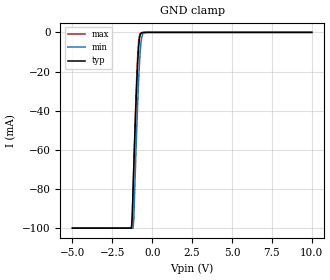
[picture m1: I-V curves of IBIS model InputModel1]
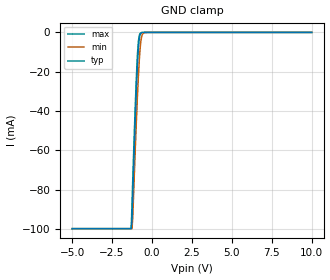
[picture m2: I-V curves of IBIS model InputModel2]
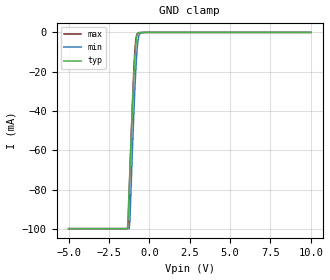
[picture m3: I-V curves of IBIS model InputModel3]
[IBIS Ver]   2.1
[File name]   pa200bv5.ibs   | pa= PSOP, f200bv= abbr chip name, 5= 5V Vcc
[File Rev]   2.00
[Date]   28-February-96
[Source]   File generated from lab measurements at Intel Corporation
[Notes]   Rev 2.00 All data was replaced by actual measurements
   performed in a lab.
[Disclaimer] INTEL DEVELOPER'S SOFTWARE LICENSE AGREEMENT
| BY USING THIS SOFTWARE, YOU ARE AGREEING TO BE BOUND
| BY THE TERMS OF THIS AGREEMENT.  DO NOT USE THE SOFTWARE
| UNTIL YOU HAVE CAREFULLY READ AND AGREED TO THE FOLLOWING
| TERMS AND CONDITIONS.  IF YOU DO NOT AGREE TO THE TERMS
| OF THIS AGREEMENT, PROMPTLY RETURN THE SOFTWARE PACKAGE
| AND ANY ACCOMPANYING ITEMS.
| IF YOU USE THIS SOFTWARE, YOU WILL BE BOUND BY THE TERMS
| OF THIS AGREEMENT
| LICENSE: Intel Corporation ("Intel") grants you the non-exclusive right
| to use the enclosed software program ("Software").  You will not use,
| copy, modify, rent, sell or transfer the Software or any portion
| thereof, except as provided in this Agreement.
| System OEM Developers may:
| 1.   Copy the Software for support, backup or archival purposes;
| 2.   Install, use, or distribute Intel owned Software in object code
|   only;
| 3.   Modify and/or use Software source code that Intel directly makes
|   available to you as an OEM Developer;
| 4.   Install, use, modify, distribute, and/or make or have made
|   derivatives ("Derivatives") of Intel owned Software under the
|   terms and conditions in this Agreement, ONLY if you are a System
|   OEM Developer and NOT an end-user.
| RESTRICTIONS:
| YOU WILL NOT:
| 1.   Copy the Software, in whole or in part, except as provided for
|   in this Agreement;
| 2.   Decompile or reverse engineer any Software provided in object
|   code format;
| 3.   Distribute any Software or Derivative code to any end-users,
|   unless approved by Intel in a prior writing.
| TRANSFER: You may transfer the Software to another OEM
| Developer if the receiving party agrees to the terms of this
| Agreement at the sole risk of any receiving party.
| OWNERSHIP AND COPYRIGHT OF SOFTWARE:
| Title to the Software and all copies thereof remain with Intel
| or its vendors.  The Software is copyrighted and is protected by
| United States and international copyright laws.  You will not
| remove the copyright notice from the Software.  You agree to
| prevent any unauthorized copying of the Software.
| DERIVATIVE WORK: OEM Developers that make or have made
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[Copyright]   Copyright 1996, Intel Corporation, All Rights Reserved
[Component]   PA28F200BV   | 44-lead PSOP package, 28F200BV
[Manufacturer]  Intel   | Boot Block (tm)
|   | operating in 5V Vcc range
[Package]
R_pkg   145.5m   144.0m   147.0m
L_pkg   5.25nH   2.00nH   8.50nH
C_pkg   1.09pF   0.68pF   1.50pF
|*****************************Pin Definitions*****************************
[Pin]   signal_name   model_name   R_pin   L_pin   C_pin
 1   VPP   POWER
 2   WP#   InputModel1
 3   NC   InputModel3
 4   A07   InputModel3
 5   A06   InputModel3
 6   A05   InputModel3
 7   A04   InputModel3
 8   A03   InputModel3
 9   A02   InputModel1
10   A01   InputModel1
11   A00   InputModel2
12   CE#   InputModel1
13   GND   GND
14   OE#   InputModel1
15   DQ0   InputOutput
16   DQ8   InputOutput
17   DQ1   InputOutput
18   DQ9   InputOutput
19   DQ2   InputOutput
20   DQ10   InputOutput
21   DQ3   InputOutput
22   DQ11   InputOutput
23   VCC   POWER
24   DQ4   InputOutput
25   DQ12   InputOutput
26   DQ5   InputOutput
27   DQ13   InputOutput
28   DQ6   InputOutput
29   DQ14   InputOutput
30   DQ7   InputOutput
31   DQ15   InputOutput
32   GND   GND
33   BYTE#   InputModel2
34   A16   InputModel2
35   A15   InputModel3
36   A14   InputModel3
37   A13   InputModel3
38   A12   InputModel3
39   A11   InputModel3
40   A10   InputModel3
41   A09   InputModel3
42   A08   InputModel3
43   WE#   InputModel1
44   RP#   InputModel1
|***********************Input Model 4******************************
[Model]   InputModel4
Model_type   Input
|   Model for all NC pins, excluding NC pin #3.
Vinl = 0.8V
Vinh = 2.0V
|Variable   Typ   Min   Max
C_comp   4.91p   NA   6.50p
[Voltage Range]   5.0V   4.5V   5.5V
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| Models and submodels in the file (5): InputModel1 (Input), InputModel2 (Input), InputModel3 (Input), InputModel4 (Input), InputOutput (I/O)
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|*********************Input Model 1************************************
[Model]   InputModel1
Model_type   Input
|   Model for WE#, WP#, RP#, OE# & CE#.
Vinl = 0.8V
Vinh = 2.0V
|Variable   Typ   Min   Max
C_comp   4.91p   NA   6.50p
[Voltage Range]   5.0V   4.5V   5.5V
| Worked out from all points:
|   GND clamp passes 1 mA (typ) near -0.74 V on its own axis
[GND_clamp]
|Voltage  I(typ)   I(min)   I(max)
-5V       -99.85mA   -99.85mA   -99.85mA
-1.3V     -99.85mA   -99.85mA   -99.85mA
-1.25V    -93.26mA   -99.85mA   -95.79mA
-1.2V     -80.3mA    -99.85mA   -81.5mA
-1.15V    -67.6mA    -94.88mA   -67.39mA
-1V       -32.49mA   -56.57mA   -29.26mA
-900mV    -13.7mA    -33.97mA   -10.19mA
-850mV    -7.324mA   -24.38mA   -4.514mA
-750mV    -1.17mA    -9.368mA   -570.4uA
-650mV    -196.9uA   -2.246mA   -163.7uA
-500mV    -19.68uA   -149.2uA   0A
10V       0A         0A         0A
[Power_clamp]
| Input buffer circuits of this product do not intrinsically
| require a [Power_clamp] definition.  This zero current
| [Power_clamp] table is provided for the compatibility with
| some IBIS parsers.
|Voltage  I(typ)   I(min)   I(max)
-5V       0A         0A         0A
0V        0A         0A         0A
5V        0A         0A         0A
10V       0A         0A         0A
|*********************Input Model 2******************************
[Model]   InputModel2
Model_type   Input
|   Model for A[0], A[16] & BYTE# pins.
Vinl = 0.8V
Vinh = 2.0V
|Variable   Typ   Min   Max
C_comp   4.91p   NA   6.50p
[Voltage Range]   5.0V   4.5V   5.5V
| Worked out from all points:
|   GND clamp passes 1 mA (typ) near -0.74 V on its own axis
[GND_clamp]
|Voltage  I(typ)   I(min)   I(max)
-5V       -99.85mA   -99.85mA   -99.85mA
-1.3V     -99.85mA   -99.85mA   -99.7mA
-1.25V    -95.1mA    -99.85mA   -86.57mA
-1.2V     -81.91mA   -93.12mA   -73.81mA
-1.05V    -44.51mA   -59.81mA   -37.94mA
-950mV    -22.91mA   -39.4mA    -17.7mA
-900mV    -14.12mA   -30.1mA    -9.812mA
-850mV    -7.485mA   -21.87mA   -4.492mA
-750mV    -1.181mA   -8.658mA   -581.8uA
-650mV    0A         -2.149mA   -166uA
-500mV    0A         -145.6uA   -18.8uA
10V       0A         0A         0A
[Power_clamp]
| Input buffer circuits of this product do not intrinsically
| require a [Power_clamp] definition.  This zero current
| [Power_clamp] table is provided for the compatibility with
| some IBIS parsers.
|Voltage  I(typ)   I(min)   I(max)
-5V       0A         0A         0A
0V        0A         0A         0A
5V        0A         0A         0A
10V       0A         0A         0A
|***********************Input Model 3******************************
[Model]   InputModel3
Model_type   Input
|   Model for A[15:1] & NC pin #3.
Vinl = 0.8V
Vinh = 2.0V
|Variable   Typ   Min   Max
C_comp   4.91p   NA   6.50p
[Voltage Range]   5.0V   4.5V   5.5V
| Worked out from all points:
|   GND clamp passes 1 mA (typ) near -0.74 V on its own axis
[GND_clamp]
|Voltage  I(typ)   I(min)   I(max)
-5V       -99.85mA   -99.86mA   -99.85mA
-1.35V    -99.85mA   -99.86mA   -99.85mA
-1.3V     -90.17mA   -99.86mA   -94.83mA
-1.25V    -79.25mA   -99.86mA   -82.83mA
-1.2V     -68.58mA   -95.57mA   -70.38mA
-1.05V    -38.07mA   -60.6mA    -36.34mA
-950mV    -20.19mA   -39.21mA   -17.09mA
-850mV    -7.009mA   -21.02mA   -4.405mA
-750mV    -1.188mA   -7.828mA   -577.2uA
-600mV    -101.4uA   -746.5uA   -94.18uA
-250mV    0A         0A         0A
10V       0A         0A         0A
[Power_clamp]
| Input buffer circuits of this product do not intrinsically
| require a [Power_clamp] definition.  This zero current
| [Power_clamp] table is provided for the compatibility with
| some IBIS parsers.
|Voltage  I(typ)   I(min)   I(max)
-5V       0A         0A         0A
0V        0A         0A         0A
5V        0A         0A         0A
10V       0A         0A         0A
